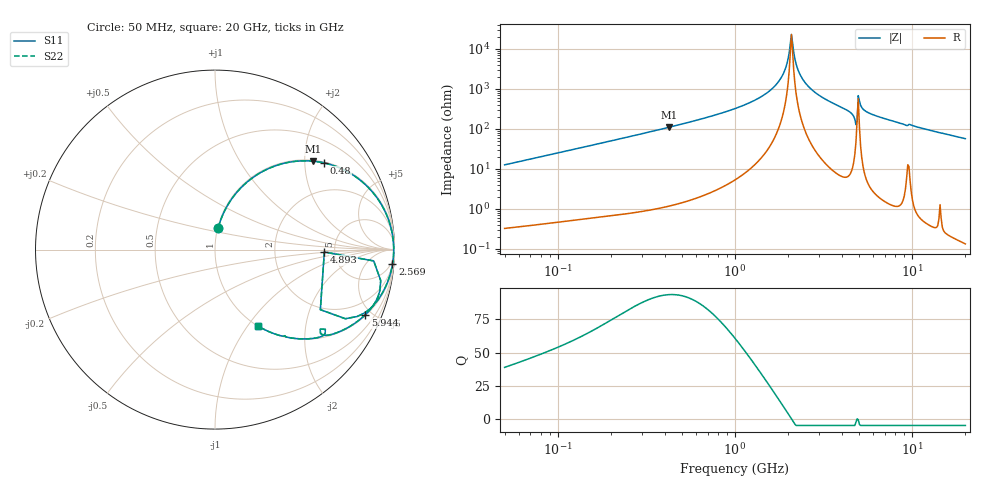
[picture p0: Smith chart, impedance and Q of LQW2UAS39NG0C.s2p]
!Murata Part Number: LQW2UAS39NG0C
!These Parameters are Measured in Series Mode Connection
!  o--[Z]--o
!Port1  Port2
!  o-------o
!Freq. Start=50[MHz] Stop=20[GHz], 401[Steps]
# Hz S RI R 50
!Freq.(Hz) S11(Real) S11(Imag) S21(Real) S21(Imag) S12(Real) S12(Imag) S22(Real) S22(Imag)
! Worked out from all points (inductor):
!   401 points, 50 MHz to 20 GHz, reference 50 ohm
!   read as one part in series: L = 39.7 nH near 51.52 MHz
!   highest Q = 93.7 at 425.8 MHz (marker M1), where L = 40.9 nH
!   self-resonance near 2.083 GHz
!   S11 on the Smith chart (normalised r, x): 50 MHz: 1.01, +0.25; 480 MHz: 1.03, +2.50; 2.569 GHz: 2, -24; 4.893 GHz: 4.11, -0.18; 5.944 GHz: 1.06, -4.58; 20 GHz: 1.00, -1.13
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5e7  0.0185 0.1225  0.9815 -0.1225  0.9815 -0.1225  0.0185 0.1225
1.364002e8  0.1072 0.3014  0.8928 -0.3014  0.8928 -0.3014  0.1072 0.3014
3.721004e8  0.4734 0.4939  0.5266 -0.4939  0.5266 -0.4939  0.4734 0.4939
4.258008e8  0.5449 0.4927  0.4551 -0.4927  0.4551 -0.4927  0.5449 0.4927
4.800071e8  0.6083 0.4828  0.3917 -0.4828  0.3917 -0.4828  0.6083 0.4828
1e9  0.9069 0.2824  0.0931 -0.2824  0.0931 -0.2824  0.9069 0.2824
1.369645e9  0.968 0.1628  0.032 -0.1628  0.032 -0.1628  0.968 0.1628
1.689197e9  0.9888 0.0816  0.0112 -0.0816  0.0112 -0.0816  0.9888 0.0816
1.904239e9  0.9944 0.0352  0.00565 -0.0352  0.00565 -0.0352  0.9944 0.0352
2.083303e9  0.9956 0.000237  0.00437 -0.000237  0.00437 -0.000237  0.9956 0.000237
2.146657e9  0.9955 -0.0114  0.00449 0.0114  0.00449 0.0114  0.9955 -0.0114
2.279204e9  0.9944 -0.0348  0.00557 0.0348  0.00557 0.0348  0.9944 -0.0348
2.569357e9  0.9889 -0.0819  0.0111 0.0819  0.0111 0.0819  0.9889 -0.0819
2.728004e9  0.9843 -0.1056  0.0157 0.1056  0.0157 0.1056  0.9843 -0.1056
4.212059e9  0.8983 -0.2924  0.1017 0.2924  0.1017 0.2924  0.8983 -0.2924
4.677679e9  0.7916 -0.3728  0.2084 0.3728  0.2084 0.3728  0.7916 -0.3728
4.89267e9  0.6091 -0.0135  0.3909 0.0135  0.3909 0.0135  0.6091 -0.0135
5.117541e9  0.9186 -0.2286  0.0814 0.2286  0.0814 0.2286  0.9186 -0.2286
5.352748e9  0.8894 -0.2992  0.1106 0.2992  0.1106 0.2992  0.8894 -0.2992
5.944466e9  0.8366 -0.3635  0.1634 0.3635  0.1634 0.3635  0.8366 -0.3635
7.442007e9  0.7301 -0.44  0.2699 0.44  0.2699 0.44  0.7301 -0.44
2e10  0.2422 -0.4273  0.7578 0.4273  0.7578 0.4273  0.2422 -0.4273
